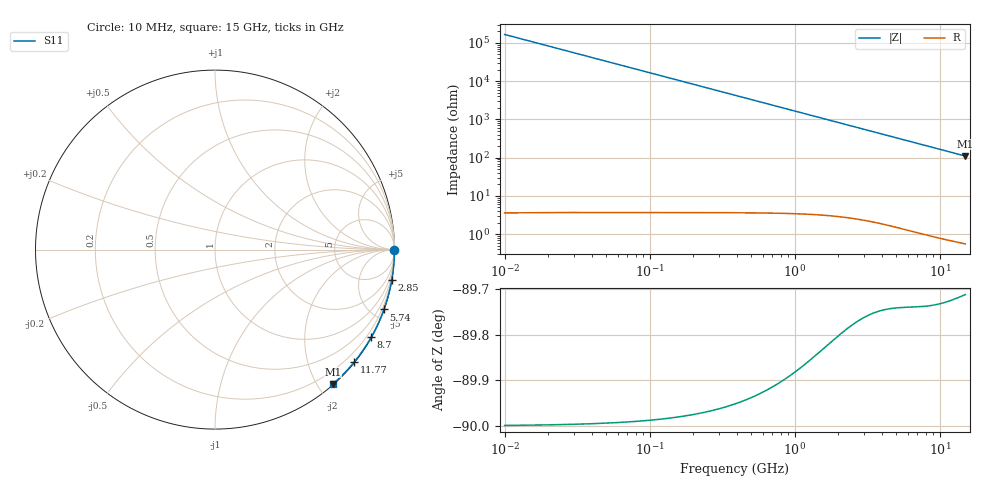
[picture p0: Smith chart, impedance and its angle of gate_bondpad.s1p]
! Created Wed Jan  6 11:08:21 2021
# hz S ma R 50
! 1 Port Network Data from SP1.SP block
! freq  magS11  angS11
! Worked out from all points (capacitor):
!   1500 points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, 10 MHz to 15 GHz, reference 50 ohm
!   read as one part to ground: C = 95.6 fF near 80 MHz
!   lowest |Z| = 110 ohm at 15 GHz (marker M1)
!   S11 on the Smith chart (normalised r, x): 10 MHz: open; 2.85 GHz: 0, -12; 5.74 GHz: 0.03, -5.82; 8.7 GHz: 0.02, -3.83; 11.77 GHz: 0.01, -2.83; 15 GHz: 0.01, -2.21
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1e7  1 -0.0
8e7  1 -0.3
5.1e8  1 -1.8
9.4e8  0.9999 -3.2
1.41e9  0.9998 -4.8
1.89e9  0.9996 -6.5
2.37e9  0.9995 -8.1
2.85e9  0.9993 -9.8
3.76e9  0.999 -12.9
4.22e9  0.9989 -14.4
4.69e9  0.9988 -16.0
5.16e9  0.9986 -17.6
5.64e9  0.9985 -19.2
5.74e9  0.9985 -19.5
6.62e9  0.9983 -22.4
7.51e9  0.998 -25.4
8.1e9  0.9979 -27.3
8.7e9  0.9977 -29.2
9.38e9  0.9976 -31.4
1.033e10  0.9973 -34.4
1.126e10  0.9971 -37.4
1.177e10  0.997 -39.0
1.245e10  0.9968 -41.1
1.313e10  0.9967 -43.1
1.366e10  0.9965 -44.7
1.419e10  0.9964 -46.3
1.489e10  0.9962 -48.4
1.5e10  0.9962 -48.7
